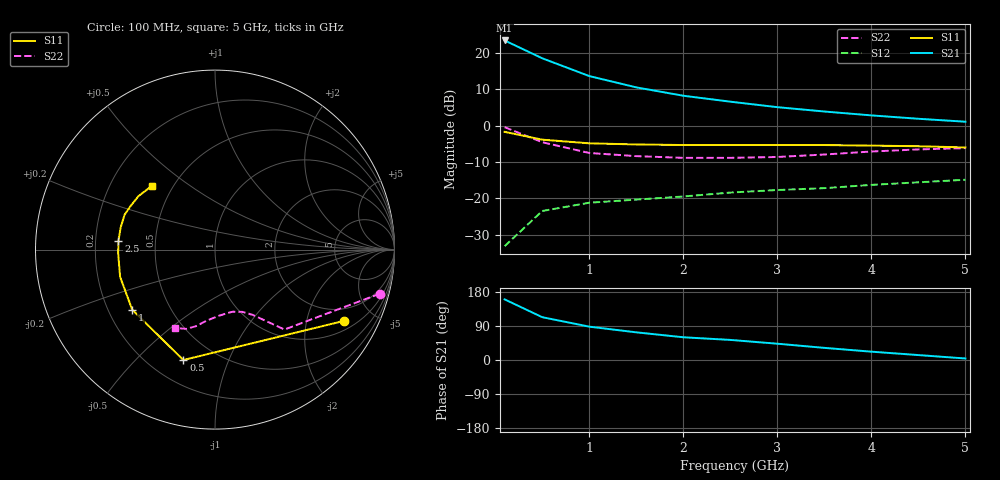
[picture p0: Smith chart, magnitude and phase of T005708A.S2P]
!AT-00570
!S-PARAMETERS at Vce=8V  Ic=5mA.  LAST UPDATED 07-21-92
!OBSOLETED Feb 1994 - nearest replacement: AT-41470
# ghz s ma r 50
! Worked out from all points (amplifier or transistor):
!   11 points, 100 MHz to 5 GHz, reference 50 ohm
!   highest |S21| = 23.4 dB at 100 MHz (marker M1)
!   |S21| within 3 dB of that: start of sweep to 345 MHz
!   unconditionally stable (mu >= 1): 1.787 GHz to end of sweep
!   at 500 MHz: K = 0.39, MSG = 21.0 dB, |S12| = -23.5 dB
!   at 2.5 GHz: K = 1.14, MAG = 10.2 dB, |S12| = -18.4 dB
!   at 5 GHz: K = 1.26, MAG = 4.9 dB, |S12| = -14.9 dB
!   S11 on the Smith chart (normalised r, x): 100 MHz: 1.38, -3.34; 500 MHz: 0.33, -0.70; 1 GHz: 0.30, -0.30; 2.5 GHz: 0.30, +0.04; 5 GHz: 0.38, +0.36
0.1  0.82 -29.0  14.78 160.0  0.022 83.0  0.95 -15.0
0.5  0.64 -106.0  8.41 113.0  0.067 40.0  0.59 -49.0
1  0.57 -144.0  4.79 88.0  0.087 33.0  0.42 -60.0
1.5  0.55 -164.0  3.35 73.0  0.096 33.0  0.38 -66.0
2  0.54 -178.0  2.57 60.0  0.106 32.0  0.36 -74.0
2.5  0.54 175.0  2.13 53.0  0.12 35.0  0.36 -78.0
3  0.54 167.0  1.79 43.0  0.13 36.0  0.37 -87.0
3.5  0.54 159.0  1.56 32.0  0.138 33.0  0.4 -97.0
4  0.53 153.0  1.38 22.0  0.153 31.0  0.44 -104.0
4.5  0.52 145.0  1.24 13.0  0.166 28.0  0.47 -110.0
5  0.5 135.0  1.13 4.0  0.18 24.0  0.49 -117.0
